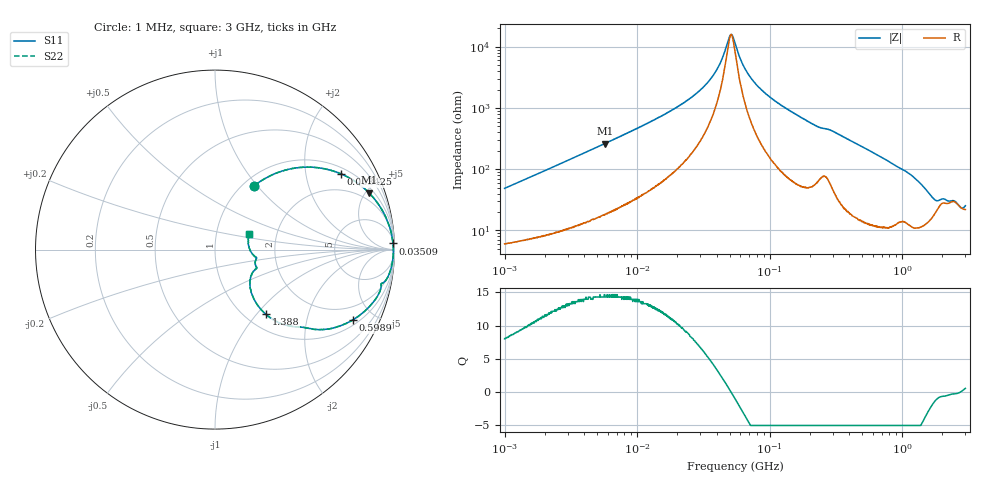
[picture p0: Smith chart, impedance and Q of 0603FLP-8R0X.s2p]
!s-Parameter Generated by FASTRON Sdn. Bhd.
!FASTRON P/N : 0603FLP-8R0X
!Keysight Technologies: E4991B_MY54100416_A.01.15
!Date: Tue Dec 02 13:10:19 2025
!Version  :Rev00  Tue Dec 02 13:10:19 2025
!Data & Calibration Information:
!Freq  S11  S21  S12  S22
!PortZ  Port1:50+j0  Port2:50+j0
!When reading reference impedance value at option line is always used.
! Remarks : This data is being provided solely for informational purposes.
# Hz S dB R 50
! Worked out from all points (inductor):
!   1601 points, 1 MHz to 3 GHz, reference 50 ohm
!   read as one part in series: L = 7.59 uH near 1.041 MHz
!   highest Q = 14.3 at 5.705 MHz (marker M1), where L = 7.32 uH
!   self-resonance near 51.07 MHz
!   S11 on the Smith chart (normalised r, x): 1 MHz: 1.12, +0.97; 3.425 MHz: 1.24, +3.17; 35.09 MHz: 12, +55; 598.9 MHz: 1.24, -3.76; 1.388 GHz: 1.23, -1.12; 3 GHz: 1.44, +0.25
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1000000  -7.57 58.4  -1.33 -24.5  -1.33 -24.5  -7.57 58.4
1945520  -3.76 44.7  -3.02 -40.2  -3.02 -40.2  -3.76 44.7
3424581  -1.73 30.9  -5.76 -54.9  -5.76 -54.9  -1.73 30.9
3804036  -1.47 28.5  -6.40 -57.3  -6.40 -57.3  -1.47 28.5
5705239  -0.78 20.3  -9.18 -65.8  -9.18 -65.8  -0.78 20.3
1.447069e7  -0.19 8.0  -17.10 -77.3  -17.10 -77.3  -0.19 8.0
2.509235e7  -0.09 3.9  -23.30 -79.3  -23.30 -79.3  -0.09 3.9
3.508696e7  -0.07 2.0  -29.10 -76.6  -29.10 -76.6  -0.07 2.0
4.201274e7  -0.06 1.0  -34.40 -68.8  -34.40 -68.8  -0.06 1.0
5.030559e7  -0.05 0.1  -43.80 -14.7  -43.80 -14.7  -0.05 0.1
5.236026e7  -0.05 -0.1  -43.70 17.2  -43.70 17.2  -0.05 -0.1
5.504702e7  -0.05 -0.4  -41.00 45.5  -41.00 45.5  -0.05 -0.4
6.493061e7  -0.06 -1.2  -33.00 72.8  -33.00 72.8  -0.06 -1.2
8.173662e7  -0.06 -2.5  -27.10 79.3  -27.10 79.3  -0.06 -2.5
1.183678e8  -0.09 -4.8  -21.40 80.3  -21.40 80.3  -0.09 -4.8
2.083556e8  -0.28 -10.0  -15.20 74.7  -15.20 74.7  -0.28 -10.0
3.798301e8  -0.57 -17.1  -10.60 69.1  -10.60 69.1  -0.57 -17.1
5.988949e8  -1.30 -27.1  -6.82 59.3  -6.82 59.3  -1.30 -27.1
7.925923e8  -2.26 -35.1  -4.78 50.2  -4.78 50.2  -2.26 -35.1
1.388188e9  -6.78 -51.8  -1.91 26.7  -1.91 26.7  -6.78 -51.8
1.818868e9  -12.10 -36.4  -1.80 10.5  -1.80 10.5  -12.10 -36.4
3e9  -13.70 24.1  -1.77 -5.9  -1.77 -5.9  -13.70 24.1
